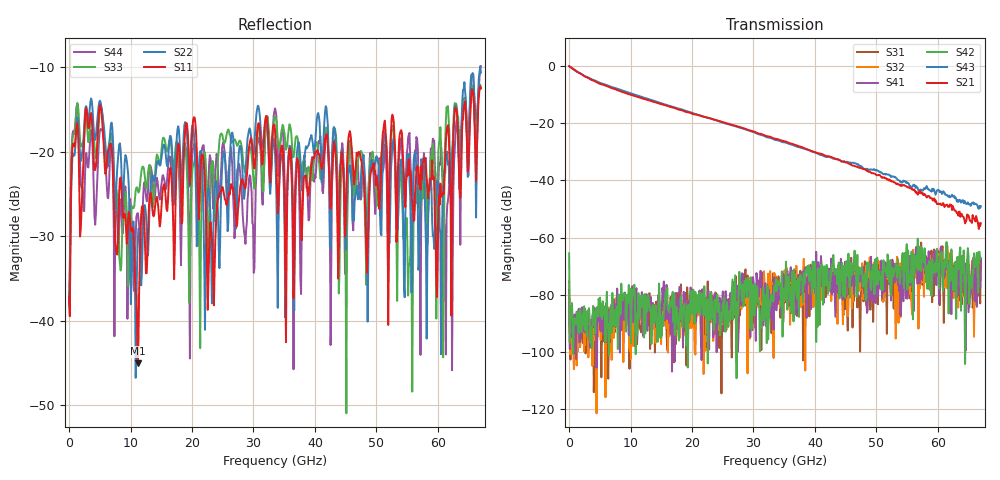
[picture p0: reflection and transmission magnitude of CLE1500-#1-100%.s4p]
!Keysight Technologies,N5247B,US50470101,A.16.20.02
!Date: Thursday, March 13, 2025 10:35:26
!Correction: S11(C  4-Port  )
!S12(C  4-Port  )
!S13(C  4-Port  )
!S14(C  4-Port  )
!S21(C  4-Port  )
!S22(C  4-Port  )
!S23(C  4-Port  )
!S24(C  4-Port  )
!S31(C  4-Port  )
!S32(C  4-Port  )
!S33(C  4-Port  )
!S34(C  4-Port  )
!S41(C  4-Port  )
!S42(C  4-Port  )
!S43(C  4-Port  )
!S44(C  4-Port  )
!S4P File: Measurements: <S11,S12,S13,S14>,
!<S21,S22,S23,S24>,
!<S31,S32,S33,S34>,
!<S41,S42,S43,S44>:
# Hz S  dB  R 50
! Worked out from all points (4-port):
!   601 points, 10 MHz to 67 GHz, reference 50 ohm
!   strongest paths, dB at 10 MHz, 16.76 GHz, 33.51 GHz, 50.25 GHz, 67 GHz:
!     S21: 0.0, -14.4, -25.4, -38.1, -55.0
!     S43: 0.0, -14.1, -25.8, -36.6, -49.0
!     S42: -65.5, -80.2, -76.6, -76.3, -67.1
!     S41: -78.3, -106.9, -76.3, -80.4, -67.5
!     S32: -75.2, -93.3, -73.4, -70.1, -71.3
!     S31: -81.7, -88.4, -84.6, -83.3, -67.6
!   lowest |S11| = -45.0 dB at 11.18 GHz (marker M1), VSWR 1.01, Z = 50.1 - j0.551 ohm
!   |S11| at or under -10 dB: start of sweep to end of sweep
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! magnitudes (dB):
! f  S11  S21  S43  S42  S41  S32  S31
! 10 MHz  -37.1  0.0  0.0  -65.5  -78.3  -75.2  -81.7
! 5.146 GHz  -14.6  -6.3  -5.9  -87.6  -92.9  -95.8  -85.7
! 11.18 GHz  -45.0  -10.8  -10.3  -89.9  -82.8  -86.3  -90.5
! 20.33 GHz  -15.9  -16.8  -16.6  -87.5  -80.2  -87.1  -84.0
! 52.71 GHz  -15.9  -40.4  -38.6  -73.6  -74.8  -73.2  -73.7
! 55.5 GHz  -22.2  -42.7  -41.9  -75.7  -66.3  -66.9  -81.4
! 67 GHz  -12.5  -55.0  -49.0  -67.1  -67.5  -71.3  -67.6
